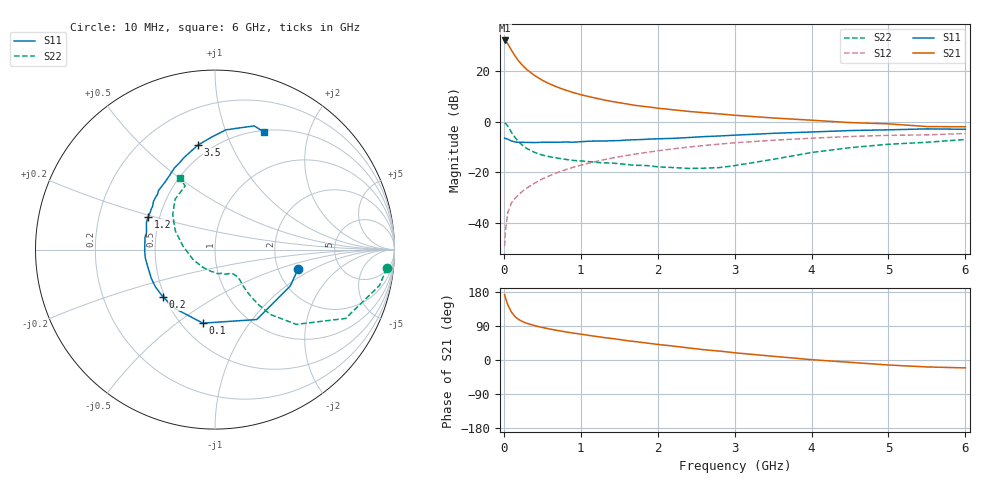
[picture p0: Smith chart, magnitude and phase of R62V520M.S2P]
! SIEMENS Small Signal Semiconductors
! BFR193
! Si NPN RF Bipolar Junction Transistor in SOT23
! VCE = 2.5 V  IC = 20 mA
! Common Emitter S-Parameters:  May  1996
# GHz  S  MA  R  50
!  f  S11  S21  S12  S22
! GHz  MAG  ANG  MAG  ANG  MAG  ANG  MAG  ANG
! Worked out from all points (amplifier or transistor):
!   36 points, 10 MHz to 6 GHz, reference 50 ohm
!   highest |S21| = 32.3 dB at 10 MHz (marker M1)
!   |S21| within 3 dB of that: start of sweep to 82.92 MHz
!   unconditionally stable (mu >= 1): 548.3 MHz to 1.879 GHz
!   at 250 MHz: K = 0.83, MSG = 24.8 dB, |S12| = -27.4 dB
!   at 1.4 GHz: K = 1.03, MAG = 10.3 dB, |S12| = -14.5 dB
!   at 6 GHz: K = 0.95, MSG = 1.3 dB, |S12| = -4.6 dB
!   lowest NFmin = 1.40 dB at 450 MHz
!   S11 on the Smith chart (normalised r, x): 10 MHz: 2.57, -0.73; 100 MHz: 0.63, -0.63; 200 MHz: 0.49, -0.30; 1.2 GHz: 0.43, +0.19; 3.5 GHz: 0.42, +0.76; 6 GHz: 0.52, +1.37
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0.01  0.475 -13.4  41.09 172.5  0.0034 87.9  0.9624 -6.2
0.02  0.4657 -25.8  40.38 165.1  0.0066 82.4  0.938 -12.3
0.05  0.4538 -59.2  35.59 146.5  0.0155 71.3  0.8225 -27.8
0.1  0.4153 -99.4  26.2 126.0  0.0248 63.0  0.6154 -42.6
0.15  0.3964 -123.5  19.73 113.5  0.0308 61.8  0.4754 -49.5
0.2  0.392 -137.8  15.6 106.0  0.0367 62.9  0.3896 -51.7
0.25  0.3914 -148.1  12.78 100.7  0.0427 64.3  0.334 -52.5
0.3  0.3896 -155.7  10.83 96.7  0.0486 65.6  0.2946 -52.7
0.4  0.3868 -166.4  8.289 90.8  0.0606 67.6  0.247 -52.1
0.5  0.3913 -173.5  6.674 85.9  0.0731 68.4  0.2185 -50.6
0.6  0.3919 -179.6  5.606 81.7  0.0858 68.8  0.2013 -51.0
0.7  0.3925 174.5  4.841 77.8  0.0986 68.7  0.1899 -50.9
0.9  0.393 166.1  3.806 71.1  0.1249 67.6  0.1709 -53.0
1.1  0.4107 158.4  3.172 65.1  0.1503 66.0  0.1622 -57.2
1.2  0.4151 154.1  2.932 62.2  0.1636 65.1  0.157 -59.2
1.7  0.44 139.3  2.126 48.7  0.2275 59.2  0.1366 -74.3
2.2  0.469 126.1  1.73 36.8  0.2902 52.3  0.1235 -99.5
2.6  0.5072 116.6  1.516 27.1  0.3378 46.5  0.1199 -127.2
3.5  0.5899 99.3  1.19 9.9  0.4298 32.6  0.1798 173.5
4.5  0.6695 84.9  0.964 -6.1  0.51 18.3  0.3063 140.3
5.5  0.7228 72.4  0.804 -18.3  0.5493 3.8  0.3917 115.1
6  0.7095 67.2  0.795 -20.9  0.5859 -0.3  0.445 116.3
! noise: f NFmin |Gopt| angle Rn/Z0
0.45  1.4  0.3  160  0.1
0.9  1.45  0.34  172  0.11
1.8  2.2  0.56  -148  0.2
